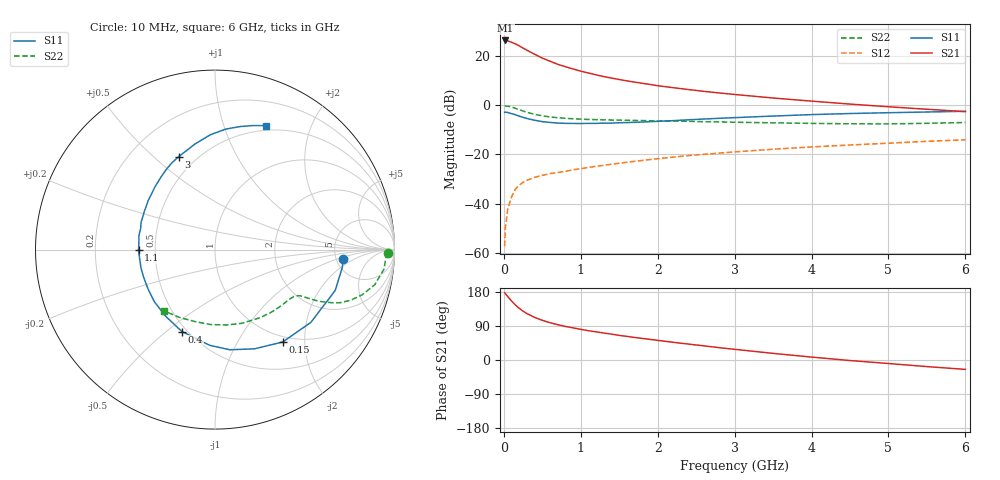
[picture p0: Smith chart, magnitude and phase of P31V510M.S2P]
! SIEMENS Small Signal Semiconductors
! BFP181
! Si NPN RF Bipolar Junction Transistor in SOT143
! VCE = 1.5 V  IC = 10 mA
! Common Emitter S-Parameters:  March  1996
# GHz  S  MA  R  50
!  f  S11  S21  S12  S22
! GHz  MAG  ANG  MAG  ANG  MAG  ANG  MAG  ANG
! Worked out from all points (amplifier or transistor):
!   36 points, 10 MHz to 6 GHz, reference 50 ohm
!   highest |S21| = 26.1 dB at 20 MHz (marker M1)
!   |S21| within 3 dB of that: start of sweep to 244.8 MHz
!   unconditionally stable (mu >= 1): 774.5 MHz to end of sweep
!   at 250 MHz: K = 0.43, MSG = 27.1 dB, |S12| = -31.2 dB
!   at 1.4 GHz: K = 1.27, MAG = 14.3 dB, |S12| = -23.9 dB
!   at 6 GHz: K = 1.11, MAG = 3.7 dB, |S12| = -14.1 dB
!   S11 on the Smith chart (normalised r, x): 10 MHz: 5.77, -1.21; 150 MHz: 0.91, -1.58; 400 MHz: 0.47, -0.57; 1.1 GHz: 0.40, -0.00; 3 GHz: 0.40, +0.60; 6 GHz: 0.45, +1.40
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0.01  0.7156 -4.1  20.12 177.5  0.0014 87.2  0.9616 -1.1
0.02  0.7164 -7.8  20.23 175.3  0.0033 93.7  0.9539 -2.6
0.05  0.7074 -18.8  19.86 167.5  0.0078 83.9  0.9476 -6.6
0.1  0.6705 -37.2  18.6 155.8  0.0139 71.2  0.9113 -12.4
0.15  0.6382 -53.8  17.25 145.2  0.0198 65.5  0.8576 -17.1
0.2  0.5949 -68.3  15.74 136.3  0.0241 60.0  0.8062 -20.5
0.25  0.5644 -81.5  14.17 128.8  0.0274 56.3  0.7572 -23.0
0.3  0.5344 -93.0  12.86 122.7  0.0301 53.3  0.7139 -24.5
0.4  0.4922 -112.0  10.64 112.4  0.0345 49.5  0.6487 -26.4
0.5  0.4618 -126.8  8.91 104.7  0.0378 46.7  0.6059 -27.2
0.6  0.4453 -139.5  7.701 98.4  0.0411 47.0  0.5754 -27.7
0.7  0.4323 -150.0  6.667 93.2  0.0432 46.9  0.5537 -28.1
0.9  0.4248 -166.1  5.37 84.8  0.0491 47.1  0.5278 -29.1
1.1  0.426 -179.6  4.447 77.3  0.0548 47.5  0.5112 -30.7
1.3  0.4311 169.6  3.761 71.1  0.0604 48.2  0.5021 -32.8
1.6  0.4419 155.6  3.084 62.3  0.0698 48.3  0.4918 -36.3
2.2  0.4837 133.8  2.244 46.7  0.0885 46.7  0.4739 -45.3
3  0.5561 111.3  1.636 28.2  0.1128 42.1  0.4488 -59.5
3.5  0.599 100.7  1.388 17.5  0.1277 38.9  0.4371 -69.8
4.5  0.674 84.9  1.046 -1.4  0.1556 31.2  0.4182 -93.4
5.5  0.7231 72.9  0.822 -17.4  0.1846 24.1  0.4269 -117.8
6  0.7475 67.6  0.736 -24.8  0.1981 19.7  0.4438 -129.9
